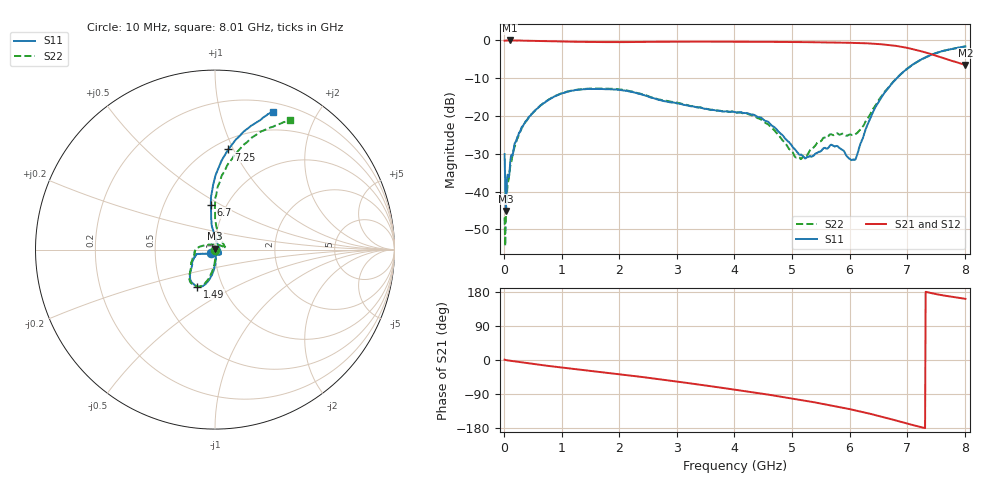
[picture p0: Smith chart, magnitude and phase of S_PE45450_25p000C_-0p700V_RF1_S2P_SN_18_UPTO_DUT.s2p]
! Device ID: PE45450
! Serial: 18
! Temp: 25.000C
! VCTRL: -0.700
! VSS: 0.000
! Control_Hi: 0.000
! Control_Lo: 0.000
! Logic State: LS_RF1
! Port 1: RF1
! Port 2: RF2
! ThroughPath:1-2
! IDD: 6.34836598e-009
! ISS: 2.59897833e-009
#  Hz  S  RI  R  50
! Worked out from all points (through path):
!   801 points, 10 MHz to 8.01 GHz, reference 50 ohm
!   highest |S21| = -0.01 dB at 100 MHz (marker M1); lowest = -6.5 dB at 8.01 GHz (marker M2)
!   group delay of S21, straight-line fit = 67.7 ps
!   lowest |S11| = -45.1 dB at 30 MHz (marker M3), VSWR 1.01, Z = 50.1 + j0.552 ohm
!   |S11| at or under -10 dB: start of sweep to 6.82 GHz
!   |S22| runs from -54.5 to -1.6 dB; largest |S21 - S12| = 0.025
!   S11 on the Smith chart (normalised r, x): 10 MHz: 0.95, -0.04; 1.49 GHz: 0.76, -0.33; 6.7 GHz: 0.85, +0.45; 7.25 GHz: 0.58, +0.95; 8.01 GHz: 0.29, +1.46
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1e7  -0.0228 -0.0215  0.9914 0.0165  0.9977 -0.00751  -0.00216 -0.004
3e7  0.000566 0.00552  0.995 -3.66e-05  1 -0.0127  0.00264 -0.00308
6e7  0.00284 -0.0165  0.9971 -0.017  0.9984 -0.0236  0.00248 -0.0114
1e8  0.00551 -0.0196  0.9979 -0.0337  0.9974 -0.0371  0.00244 -0.0196
2.4e8  0.00258 -0.0538  0.991 -0.0833  0.9934 -0.0867  0.00061 -0.0514
4.8e8  -0.0047 -0.1064  0.9739 -0.1698  0.9749 -0.1706  -0.00989 -0.1055
8.7e8  -0.0384 -0.1764  0.9277 -0.293  0.9281 -0.2946  -0.0448 -0.1755
1.35e9  -0.0863 -0.2082  0.8584 -0.4213  0.8584 -0.4207  -0.0931 -0.2064
1.49e9  -0.0982 -0.2056  0.8368 -0.4564  0.8374 -0.4558  -0.104 -0.2048
2.11e9  -0.1381 -0.1664  0.7329 -0.6043  0.7337 -0.604  -0.1426 -0.167
2.68e9  -0.1302 -0.0986  0.6113 -0.7393  0.6116 -0.7384  -0.1335 -0.0985
4.01e9  -0.1079 -0.0316  0.1941 -0.9412  0.1939 -0.9408  -0.112 -0.00998
4.57e9  -0.0816 -0.0228  -0.0163 -0.957  -0.0165 -0.9563  -0.0767 0.0182
5.08e9  -0.0223 -0.0256  -0.2223 -0.9255  -0.2218 -0.9246  -0.00482 0.0279
5.35e9  0.00669 -0.0284  -0.3331 -0.8861  -0.3329 -0.8857  0.0288 0.0236
5.7e9  0.033 -0.0244  -0.4757 -0.8088  -0.4746 -0.8092  0.0552 0.0119
6.08e9  0.0204 0.0169  -0.6233 -0.6864  -0.6231 -0.6856  0.0415 0.0378
6.41e9  -0.0123 0.1139  -0.7327 -0.5333  -0.7322 -0.5329  0.00838 0.1245
6.68e9  -0.0232 0.2376  -0.7847 -0.3747  -0.7838 -0.3749  -5.2e-05 0.2413
6.7e9  -0.023 0.2484  -0.7872 -0.3622  -0.786 -0.3628  0.000453 0.2528
7.25e9  0.074 0.5577  -0.7148 -0.0315  -0.7147 -0.0324  0.1256 0.5458
8.01e9  0.322 0.7668  -0.4467 0.1501  -0.4472 0.1492  0.4172 0.7207
